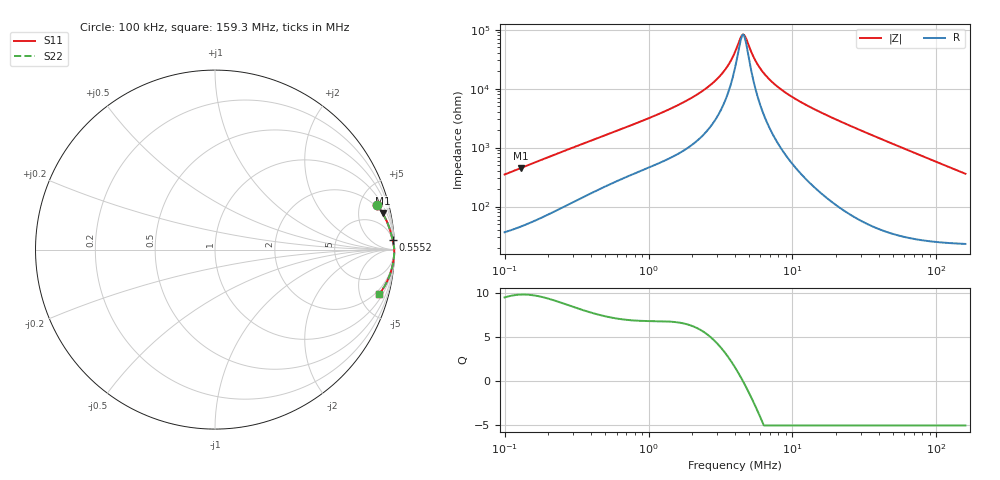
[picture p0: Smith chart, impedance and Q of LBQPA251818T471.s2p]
! LBQPA251818T471  S-PARAMETER MODEL  ( General Type )
! Model Generated by TAIYO YUDEN Corporation (http://www.ty-top.com)
! Version 1.0
! TAIYO YUDEN Control No. 191025NI43SB-FBB
! Copyright(c) 2019 TAIYO YUDEN CO.,LTD. All Rights Reserved.
! Product Description (link to TY-COMPAS)
! https://ds.yuden.co.jp/TYCOMPAS/or/detail?pn=LBQPA251818T471K&u=M
! Products Name : Inductors
! Characteristics :
!  Inductance : 470 uH , SRF(min) : 3.5 MHz , DC Resistance(max) : 28.6 Ohm
!  Rated Current : Saturation :80 mA , Temp Rise : 50 mA (20 degC)
!  Case Size : 2.5 x 1.8 / 0.098 x 0.071 [mm/inch] , Thickness : 1.8 / 0.071 [mm/inch]
!  (Conditions: Temperature = 25 degC , DC Bias Current/Voltage = 0A / 0V)
! External Node Assignments :
!  1  o---GGG---o  2
! GND o---------o GND
! Frequency Range : 0.1MHz  -  159.254811MHz  [ 402 STEP ]
# MHz S RI R 50
! Freq[MHz].  S11 Real  S11 Imag  S21 Real  S21 Imag  S12 Real  S12 Imag  S22 Real  S22 Imag
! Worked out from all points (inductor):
!   401 points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, 100 kHz to 159.3 MHz, reference 50 ohm
!   read as one part in series: L = 549 uH near 103.8 kHz
!   highest Q = 9.8 at 129.4 kHz (marker M1), where L = 549 uH
!   self-resonance near 4.457 MHz
!   S11 on the Smith chart (normalised r, x): 100 kHz: 1.73, +6.93; 555.2 kHz: 6, +35; 159.3 MHz: 1.46, -7.17
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0.1  0.9016 0.2497  0.0984 -0.2497  0.0984 -0.2497  0.9016 0.2497
0.129441  0.934 0.2024  0.066 -0.2024  0.066 -0.2024  0.934 0.2024
0.343835  0.9821 0.0844  0.0179 -0.0844  0.0179 -0.0844  0.9821 0.0844
0.555247  0.9893 0.0545  0.0107 -0.0545  0.0107 -0.0545  0.9893 0.0545
1.182227  0.9954 0.0263  0.00459 -0.0263  0.00459 -0.0263  0.9954 0.0263
1.909137  0.9974 0.015  0.00258 -0.015  0.00258 -0.015  0.9974 0.015
2.709795  0.9982 0.00837  0.00176 -0.00837  0.00176 -0.00837  0.9982 0.00837
3.443534  0.9986 0.00437  0.00143 -0.00437  0.00143 -0.00437  0.9986 0.00437
3.775988  0.9987 0.0029  0.00134 -0.0029  0.00134 -0.0029  0.9987 0.0029
4.064915  0.9987 0.00173  0.00128 -0.00173  0.00128 -0.00173  0.9987 0.00173
4.375951  0.9988 0.000567  0.00123 -0.000567  0.00123 -0.000567  0.9988 0.000567
4.540283  0.9988 -1.34e-05  0.00121 1.34e-05  0.00121 1.34e-05  0.9988 -1.34e-05
4.624749  0.9988 -0.000304  0.0012 0.000304  0.0012 0.000304  0.9988 -0.000304
4.798424  0.9988 -0.000885  0.00118 0.000885  0.00118 0.000885  0.9988 -0.000885
5.261684  0.9989 -0.00235  0.00114 0.00235  0.00114 0.00235  0.9989 -0.00235
5.664293  0.9989 -0.00353  0.00112 0.00353  0.00112 0.00353  0.9989 -0.00353
6.810798  0.9989 -0.0066  0.0011 0.0066  0.0011 0.0066  0.9989 -0.0066
9.147063  0.9988 -0.012  0.00117 0.012  0.00117 0.012  0.9988 -0.012
13.72135  0.9985 -0.0213  0.00151 0.0213  0.00151 0.0213  0.9985 -0.0213
47.17884  0.991 -0.0809  0.009 0.0809  0.009 0.0809  0.991 -0.0809
95.04868  0.9668 -0.1593  0.0332 0.1593  0.0332 0.1593  0.9668 -0.1593
159.2548  0.9143 -0.2494  0.0857 0.2494  0.0857 0.2494  0.9143 -0.2494
